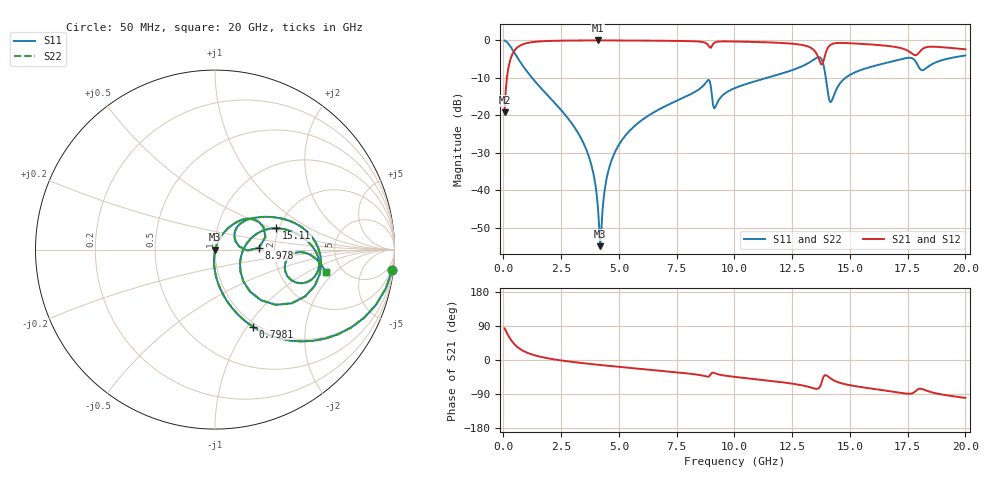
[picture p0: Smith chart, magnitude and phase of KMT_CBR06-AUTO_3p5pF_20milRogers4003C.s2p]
! Data measured by Modelithics Inc. support@modelithics.com 813-866-6335
! KEMET CBR06-AUTO 3.5pF, Pad Width= 0.851mm, Pad Length= 0.64mm, Pad Gap= 0.62mm, 20mil Rogers 4003C substrate Data, January 2022
# hz S ma R 50
! 2 Port Network Data from SP1.SP block
! freq  magS11  angS11  magS21  angS21  magS12  angS12  magS22  angS22
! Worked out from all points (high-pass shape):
!   401 points, 50 MHz to 20 GHz, reference 50 ohm
!   highest |S21| = -0.02 dB at 4.09 GHz (marker M1); lowest = -19.2 dB at 50 MHz (marker M2)
!   |S21| within 3 dB of the highest: 446.1 MHz to 13.5 GHz (13.05 GHz wide, 187 % of centre); 13.97 GHz to 17.58 GHz (3.606 GHz wide, 22.9 % of centre)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
!   lowest |S11| = -54.9 dB at 4.19 GHz (marker M3), VSWR 1.00, Z = 50.2 - j0.0647 ohm
!   |S11| at or under -10 dB: 1.238 GHz to 11.4 GHz (10.16 GHz wide, 161 % of centre); 13.96 GHz to 14.81 GHz (851.7 MHz wide, 5.92 % of centre)
!   |S22| runs from -54.9 to -0.1 dB; largest |S21 - S12| = 0
!   S11 on the Smith chart (normalised r, x): 50 MHz: 1, -18; 798.1 MHz: 0.96, -1.06; 8.978 GHz: 1.65, +0.04; 15.11 GHz: 1.94, +0.53; 20 GHz: 3.73, -1.54
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5e7  0.9939 -6.5  0.1103 83.5  0.1103 83.5  0.9939 -6.5
2.99375e8  0.8314 -34.6  0.5549 55.3  0.5549 55.3  0.8314 -34.6
7.98125e8  0.4783 -63.8  0.8772 26.1  0.8772 26.1  0.4783 -63.8
3.391625e9  0.04733 -96.0  0.9971 -8.0  0.9971 -8.0  0.04733 -96.0
3.8405e9  0.01977 -96.0  0.998 -11.0  0.998 -11.0  0.01977 -96.0
4.089875e9  0.005922 -85.3  0.9981 -12.6  0.9981 -12.6  0.005922 -85.3
4.189625e9  0.001796 -21.0  0.9981 -13.2  0.9981 -13.2  0.001796 -21.0
4.488875e9  0.01551 68.2  0.9979 -15.0  0.9979 -15.0  0.01551 68.2
4.887875e9  0.03523 69.5  0.9973 -17.4  0.9973 -17.4  0.03523 69.5
6.73325e9  0.1198 60.8  0.9901 -28.0  0.9901 -28.0  0.1198 60.8
8.828e9  0.2891 32.3  0.8903 -43.9  0.8903 -43.9  0.2891 32.3
8.977625e9  0.246 2.5  0.7976 -37.1  0.7976 -37.1  0.246 2.5
9.177125e9  0.1298 33.2  0.9455 -35.6  0.9455 -35.6  0.1298 33.2
1.0025e10  0.2313 43.9  0.9664 -44.6  0.9664 -44.6  0.2313 43.9
1.336662e10  0.5366 8.9  0.7751 -73.5  0.7751 -73.5  0.5366 8.9
1.38155e10  0.5218 -35.0  0.4875 -51.0  0.4875 -51.0  0.5218 -35.0
1.416462e10  0.1496 -13.3  0.8738 -48.7  0.8738 -48.7  0.1496 -13.3
1.511225e10  0.3614 19.2  0.9131 -67.8  0.9131 -67.8  0.3614 19.2
1.670825e10  0.5128 5.7  0.8389 -82.2  0.8389 -82.2  0.5128 5.7
1.785538e10  0.5185 -21.2  0.6353 -81.5  0.6353 -81.5  0.5185 -21.2
1.850375e10  0.4712 -1.7  0.8241 -84.5  0.8241 -84.5  0.4712 -1.7
2e10  0.6301 -11.4  0.7609 -100.1  0.7609 -100.1  0.6301 -11.4
